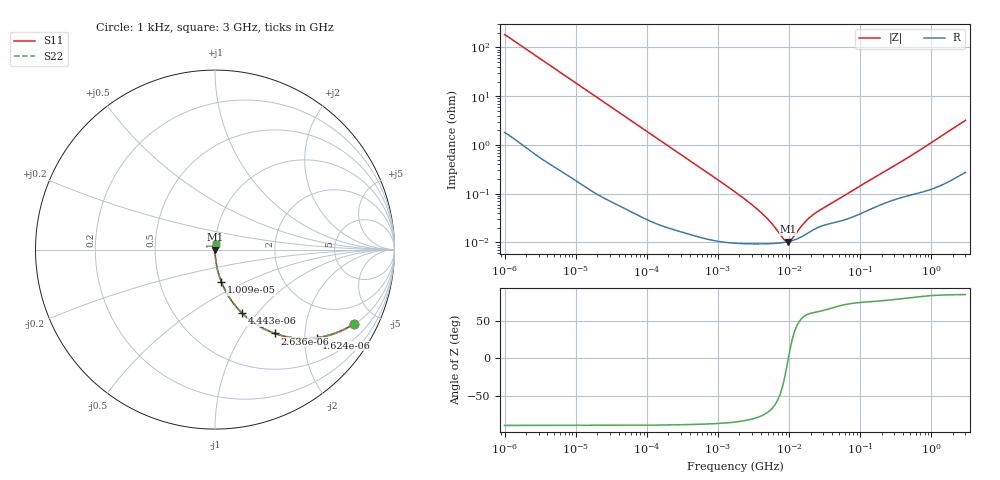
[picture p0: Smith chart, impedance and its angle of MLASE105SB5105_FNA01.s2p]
! MLASE105SB5105_FNA01  S-PARAMETER MODEL  ( Standard Model )
! Model Generated by TAIYO YUDEN Corporation (http://www.ty-top.com)
! Version 1.0
! TAIYO YUDEN Control No. 220601
! Copyright(c) 2009 TAIYO YUDEN CO.,LTD. All Rights Reserved.
! Product Description (link to TY-COMPAS)
! https://ds.yuden.co.jp/TYCOMPAS/or/detail?pn=MLASE105SB5105KFNA01&u=M
! Products Name : Multilayer Ceramic Capacitors
! Characteristics :
!  Capacitance : 1 [uF] , Rated Voltage : 16 [V] , TCC : X5R
!  Case Size : 1.0 x 0.5 / 0.039 x 0.02 [mm/inch] , Thickness : 0.5 / 0.02 [mm/inch]
!  (Conditions: Temperature = 25 [degC] , DC Bias Voltage = 0 [V])
! External Node Assignments :
!  1  o---| |---o  2
! GND o---------o GND
! Frequency Range : 1kHz  -  3GHz  [ 401 STEP ]
# MHZ S RI R 50
! Freq[MHz].  S11 Real  S11 Imag  S21 Real  S21 Imag  S12 Real  S12 Imag  S22 Real  S22 Imag
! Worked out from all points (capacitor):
!   401 points, 1 kHz to 3 GHz, reference 50 ohm
!   read as one part in series: C = 858 nF near 1.077 kHz
!   lowest |Z| = 10.4 mohm at 9.626 MHz (marker M1)
!   series resonance near 9.736 MHz, so ESL is about 310 pH
!   S11 on the Smith chart (normalised r, x): 1 kHz: 1.04, -3.70; 1.624 kHz: 1.02, -2.29; 2.636 kHz: 1.01, -1.41; 4.443 kHz: 1.01, -0.84; 10.09 kHz: 1.00, -0.37; 3 GHz: 1.01, +0.06
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0.001  0.7717 -0.4149  0.2283 0.4149  0.2283 0.4149  0.7717 -0.4149
0.001624  0.5661 -0.4908  0.4339 0.4908  0.4339 0.4908  0.5661 -0.4908
0.002031  0.4565 -0.4934  0.5435 0.4934  0.5435 0.4934  0.4565 -0.4934
0.002636  0.3344 -0.4672  0.6656 0.4672  0.6656 0.4672  0.3344 -0.4672
0.004443  0.1525 -0.3548  0.8475 0.3548  0.8475 0.3548  0.1525 -0.3548
0.006451  0.0798 -0.2662  0.9202 0.2662  0.9202 0.2662  0.0798 -0.2662
0.010091  0.0351 -0.1791  0.9649 0.1791  0.9649 0.1791  0.0351 -0.1791
0.01216  0.0247 -0.1505  0.9753 0.1505  0.9753 0.1505  0.0247 -0.1505
0.033275  0.00386 -0.0565  0.9961 0.0565  0.9961 0.0565  0.00386 -0.0565
0.147855  0.000397 -0.0129  0.9996 0.0129  0.9996 0.0129  0.000397 -0.0129
1.732051  9.77e-05 -0.00109  0.9999 0.00109  0.9999 0.00109  9.77e-05 -0.00109
4.083148  9.37e-05 -0.000393  0.9999 0.000393  0.9999 0.000393  9.37e-05 -0.000393
5.711239  9.5e-05 -0.000224  0.9999 0.000224  0.9999 0.000224  9.5e-05 -0.000224
8.291982  9.98e-05 -6.48e-05  0.9999 6.48e-05  0.9999 6.48e-05  9.98e-05 -6.48e-05
8.933959  0.000102 -3.46e-05  0.9999 3.46e-05  0.9999 3.46e-05  0.000102 -3.46e-05
9.625639  0.000104 -4.53e-06  0.9999 4.53e-06  0.9999 4.53e-06  0.000104 -4.53e-06
10.76485  0.000108 4.05e-05  0.9999 -4.05e-05  0.9999 -4.05e-05  0.000108 4.05e-05
15.62917  0.000136 0.000193  0.9999 -0.000193  0.9999 -0.000193  0.000136 0.000193
21.06097  0.000176 0.000313  0.9998 -0.000313  0.9998 -0.000313  0.000176 0.000313
27.34186  0.000212 0.000414  0.9998 -0.000414  0.9998 -0.000414  0.000212 0.000414
256.0921  0.000703 0.00318  0.9993 -0.00318  0.9993 -0.00318  0.000703 0.00318
3000  0.00374 0.0317  0.9963 -0.0317  0.9963 -0.0317  0.00374 0.0317
